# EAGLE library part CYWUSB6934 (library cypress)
WirelessUSB LS 2.4 GHz DSSS Radio SoC Source: http://v4.cypress.com/cfuploads/img/products/cywusb6934.pdf
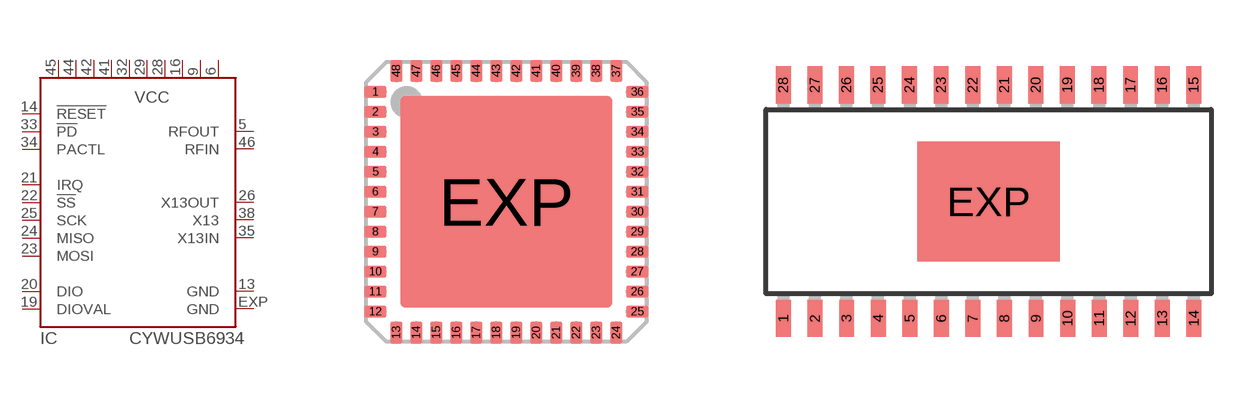
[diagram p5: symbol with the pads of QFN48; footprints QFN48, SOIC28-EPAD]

Designator prefix IC

## CYWUSB6934-48LFG (OC_FARNELL: unknown; OC_NEWARK: unknown)  [QFN48]
5  RFOUT  out
6  VCC  pwr
9  VCC  pwr
13  GND  pwr
14  !RESET  in
16  VCC  pwr
19  DIOVAL
20  DIO
21  IRQ  hiz
22  !SS  in
23  MOSI  in
24  MISO  hiz
25  SCK  in
26  X13OUT  out
28  VCC  pwr
29  VCC  pwr
32  VCC  pwr
33  !PD  in
34  PACTL
35  X13IN  in
38  X13  in
41  VCC  pwr
42  VCC  pwr
44  VCC  pwr
45  VCC  pwr
46  RFIN  in
EXP  GND  pwr

## CYWUSB6934-SE28 (OC_FARNELL: unknown; OC_NEWARK: unknown)  [SOIC28-EPAD]
1  VCC  pwr
2  VCC  pwr
3  RFIN  in
6  RFOUT  out
7  VCC  pwr
8  VCC  pwr
9  GND  pwr
10  !RESET  in
11  VCC  pwr
12  DIOVAL
13  DIO
14  IRQ  hiz
15  !SS  in
16  MOSI  in
17  MISO  hiz
18  SCK  in
19  X13OUT  out
20  VCC  pwr
21  VCC  pwr
22  VCC  pwr
23  !PD  in
24  PACTL
25  X13IN  in
26  X13  in
27  VCC  pwr
28  VCC  pwr
EXP  GND  pwr

## Footprint QFN48 (pad centres in mm)
48-pin QFN 7 x 7 mm LF48 48 Quad Flat Package No Leads Source: http://v4.cypress.com/cfuploads/img/products/cywusb6934.pdf
smd 0.55 x 0.3: 1 -3.275,2.75; 2 -3.275,2.25; 3 -3.275,1.75; 4 -3.275,1.25; 5 -3.275,0.75; 6 -3.275,0.25; 7 -3.275,-0.25; 8 -3.275,-0.75; 9 -3.275,-1.25; 10 -3.275,-1.75; 11 -3.275,-2.25; 12 -3.275,-2.75; 25 3.275,-2.75; 26 3.275,-2.25; 27 3.275,-1.75; 28 3.275,-1.25; 29 3.275,-0.75; 30 3.275,-0.25; 31 3.275,0.25; 32 3.275,0.75; 33 3.275,1.25; 34 3.275,1.75; 35 3.275,2.25; 36 3.275,2.75
smd 0.3 x 0.55: 13 -2.75,-3.275; 14 -2.25,-3.275; 15 -1.75,-3.275; 16 -1.25,-3.275; 17 -0.75,-3.275; 18 -0.25,-3.275; 19 0.25,-3.275; 20 0.75,-3.275; 21 1.25,-3.275; 22 1.75,-3.275; 23 2.25,-3.275; 24 2.75,-3.275; 37 2.75,3.275; 38 2.25,3.275; 39 1.75,3.275; 40 1.25,3.275; 41 0.75,3.275; 42 0.25,3.275; 43 -0.25,3.275; 44 -0.75,3.275; 45 -1.25,3.275; 46 -1.75,3.275; 47 -2.25,3.275; 48 -2.75,3.275
smd 5.309 x 5.309: EXP 0,0

## Footprint SOIC28-EPAD (pad centres in mm)
28-pin (300-Mil) SOIC EPAD SE28.3 Source: http://v4.cypress.com/cfuploads/img/products/cywusb6934.pdf
smd 0.6 x 1.5: 1 -8.25,-4.7; 2 -6.98,-4.7; 3 -5.71,-4.7; 4 -4.44,-4.7; 5 -3.17,-4.7; 6 -1.9,-4.7; 7 -0.63,-4.7; 8 0.64,-4.7; 9 1.91,-4.7; 10 3.18,-4.7; 11 4.45,-4.7; 12 5.72,-4.7; 13 6.99,-4.7; 14 8.26,-4.7; 15 8.25,4.7; 16 6.98,4.7; 17 5.71,4.7; 18 4.44,4.7; 19 3.17,4.7; 20 1.9,4.7; 21 0.63,4.7; 22 -0.64,4.7; 23 -1.91,4.7; 24 -3.18,4.7; 25 -4.45,4.7; 26 -5.72,4.7; 27 -6.99,4.7; 28 -8.26,4.7
smd 5.715 x 4.826: EXP 0,0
